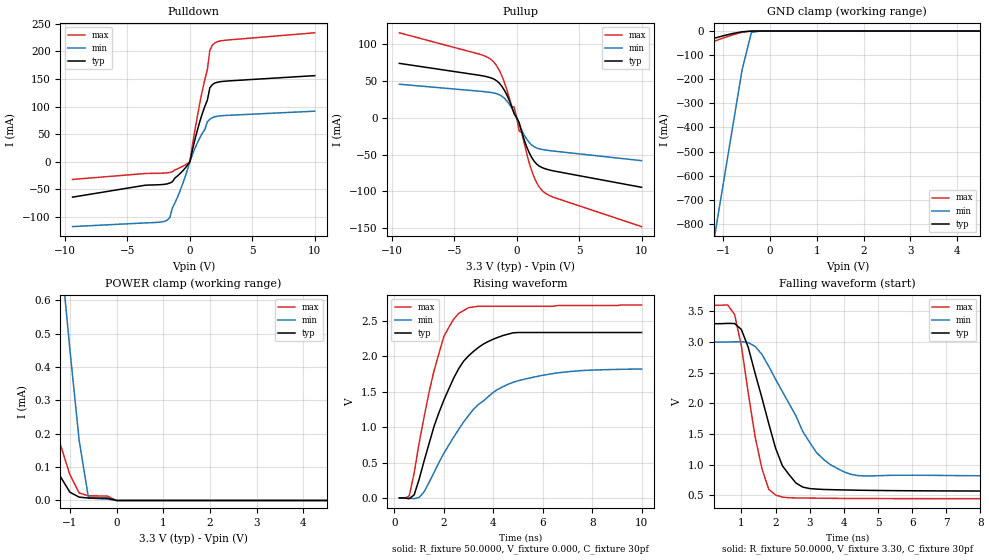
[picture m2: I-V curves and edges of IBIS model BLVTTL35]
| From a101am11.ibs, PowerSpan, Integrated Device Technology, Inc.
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|   Model LVTTL tristate_driver
[Model]   BLVTTL35
Model_type   I/O
Polarity   Non-Inverting
Enable   Active-High
Vinl = 1.16v
Vinh = 1.65v
C_comp   10.5pf   8pf   12pf
[Temperature Range]   27.0   125.0   -40.0
[Pullup Reference]   3.30V   3.00V   3.60V
[Pulldown Reference]   0.00V   0.00V   0.00V
[POWER Clamp Reference]   3.30V   3.00V   3.60V
[GND Clamp Reference]   0.00V   0.00V   0.00V
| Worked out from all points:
|   slope of the pulldown table from 0 to 0.495 V, typ, clamps not added: 10.3 ohm
|   slope of the pullup table from 0 to 0.495 V, typ, clamps not added: 20.4 ohm
|   GND clamp passes 1 mA (typ) near -0.46 V on its own axis
|   POWER clamp passes 1 mA (typ) near -2.40 V on its own axis
|   rising waveform, R_fixture 50.0000, V_fixture 0.000, C_fixture 30pf: 20-80 % time 1.52ns typ, 2.27ns min, 1.03ns max; typ from 0 V to 2.34 V
|   falling waveform, R_fixture 50.0000, V_fixture 3.30, C_fixture 30pf: 20-80 % time 832ps typ, 1.3ns min, 560ps max; typ from 3.3 V to 0.569 V
[Pulldown]
|   volt   I(typ)   I(min)   I(max)
-9.4V     -64.1mA    -117.5mA   -32.05mA
-2V       -40.79mA   -107.8mA   -20.39mA
-1.6V     -38.51mA   -101mA     -19.25mA
-1.4V     -36.32mA   -83.47mA   -18.16mA
-400mV    -12.04mA   -28.56mA   -6.02mA
0V        0A         0A         0A
800mV     73.21mA    43.5mA     106.8mA
1.4V      111.6mA    72.65mA    166.9mA
1.6V      134.1mA    77.01mA    201.9mA
1.8V      139.8mA    79.92mA    211.2mA
2.8V      146mA      83.84mA    220.2mA
10V       156.1mA    91.66mA    233.7mA
[Pullup]
|volt  I(typ)   I(min)   I(max)
-9.4V     74.06mA    45.7mA     115.6mA
-2V       53.92mA    34.29mA    78.58mA
-1.4V     47.24mA    31.54mA    64.75mA
-1V       37.89mA    26.78mA    48.87mA
-400mV    15.3mA     13.37mA    15.86mA
-200mV    5.405mA    7.143mA    14.41mA
200mV     -6.756mA   -8.928mA   -18.01mA
400mV     -19.13mA   -16.72mA   -19.83mA
1.2V      -53.9mA    -36.95mA   -71.89mA
2V        -67.4mA    -42.86mA   -98.22mA
3V        -72.36mA   -45.27mA   -108.3mA
10V       -94.47mA   -58.23mA   -147.9mA
[GND_clamp]
|volt   I(typ)   I(min)   I(max)
-9.4V     -538.8mA   -10.44A    -659mA
-1.2V     -30.17mA   -864.3mA   -42.9mA
-1V       -19.52mA   -629.5mA   -28.74mA
-600mV    -3.127mA   -161.4mA   -5.345mA
-400mV    -184.9uA   -5.554mA   -308.8uA
-200mV    -9.882uA   -33.14uA   -16.07uA
10V       0A         0A         0A
[POWER_clamp]
|volt   I(typ)   I(min)   I(max)
-9.4V     343.3mA    202.4mA    484.6mA
-2.6V     153.1mA    2.753mA    237.6mA
-2.4V     237.5uA    2.432mA    371.5uA
-2V       159.1uA    1.887mA    276uA
-1.6V     83.41uA    1.282mA    272uA
-1.4V     80uA       996.6uA    269.2uA
-1.2V     71.48uA    751.2uA    166.9uA
-1V       25.15uA    454.8uA    78.12uA
-800mV    10.05uA    180.6uA    22.62uA
-600mV    7.328uA    7.772uA    13.93uA
0V        0A         0A         0A
10V       0A         0A         0A
[Ramp]
| variable   typ   min   max
dV/dt_r   1.41/1.60ns   1.10/2.20ns   1.65/1.00ns
dV/dt_f   1.98/0.80ns   1.80/1.20ns   2.16/0.60ns
R_load = 100.0000
[Rising Waveform]
R_fixture = 50.0000
V_fixture = 0.000
C_fixture = 30pf
| time   V(typ)   V(min)   V(max)
200ps     341.4uV    290.8uV    407.3uV
600ps     -10.51mV   -3.992mV   28.73mV
800ps     44.76mV    -10.14mV   354.7mV
1.2ns     522.4mV    85.69mV    1.144V
1.6ns     1.009V     356.6mV    1.795V
2ns       1.383V     630.7mV    2.283V
2.6ns     1.827V     968.4mV    2.609V
3.6ns     2.176V     1.371V     2.71V
4.8ns     2.334V     1.635V     2.71V
10ns      2.339V     1.822V     2.729V
[Falling Waveform]
R_fixture = 50.0000
V_fixture = 3.30
V_fixture_min = 3.00
V_fixture_max = 3.60
C_fixture = 30pf
| time   V(typ)   V(min)   V(max)
200ps     3.3V       3V         3.6V
800ps     3.303V     3.005V     3.452V
1.2ns     2.915V     2.992V     2.171V
1.6ns     2.093V     2.801V     938.9mV
2ns       1.272V     2.394V     505.4mV
2.2ns     983.5mV    2.193V     471.3mV
2.8ns     634.2mV    1.539V     456.9mV
3.4ns     596.4mV    1.089V     452.6mV
4.2ns     586.2mV    844.7mV    449.3mV
13.8ns    568.8mV    809.1mV    445.6mV
